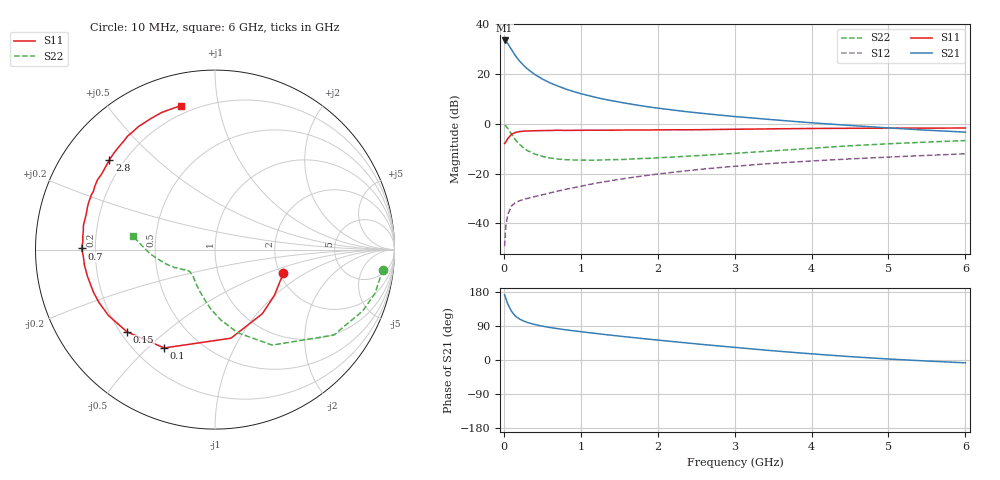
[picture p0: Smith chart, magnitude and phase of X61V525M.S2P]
! SIEMENS Small Signal Semiconductors
! BFP193W
! Si NPN RF Bipolar Junction Transistor in SOT343
! VCE = 1.5 V  IC = 25 mA
! Common Emitter S-Parameters:  April 1994
# GHz  S  MA  R  50
!  f  S11  S21  S12  S22
! GHz  MAG  ANG  MAG  ANG  MAG  ANG  MAG  ANG
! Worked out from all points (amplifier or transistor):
!   40 points, 10 MHz to 6 GHz, reference 50 ohm
!   highest |S21| = 33.5 dB at 10 MHz (marker M1)
!   |S21| within 3 dB of that: start of sweep to 86.36 MHz
!   unconditionally stable (mu >= 1): 783.3 MHz to 4.294 GHz
!   at 200 MHz: K = 0.42, MSG = 28.1 dB, |S12| = -30.9 dB
!   at 1.5 GHz: K = 1.14, MAG = 13.3 dB, |S12| = -22.3 dB
!   at 6 GHz: K = 0.96, MSG = 4.4 dB, |S12| = -12.0 dB
!   S11 on the Smith chart (normalised r, x): 10 MHz: 2.09, -0.66; 100 MHz: 0.32, -0.56; 150 MHz: 0.23, -0.38; 700 MHz: 0.15, +0.00; 2.8 GHz: 0.15, +0.36; 6 GHz: 0.16, +0.78
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0.01  0.4028 -19.1  47.2 172.3  0.0035 86.1  0.9415 -6.8
0.02  0.4178 -37.6  46.48 166.3  0.0068 78.4  0.924 -15.4
0.03  0.444 -53.5  45.17 159.9  0.0098 72.4  0.8912 -22.5
0.05  0.5016 -79.8  41.16 148.2  0.015 63.4  0.8154 -35.7
0.1  0.6167 -117.3  30.9 128.2  0.0224 48.8  0.6202 -59.1
0.15  0.6711 -136.9  23.45 116.0  0.0263 42.0  0.4806 -74.7
0.2  0.6976 -148.1  18.54 108.6  0.0284 39.5  0.3929 -85.3
0.25  0.7104 -155.4  15.3 103.4  0.0302 39.0  0.3364 -93.4
0.3  0.7177 -160.7  12.9 99.6  0.0316 39.0  0.2948 -99.9
0.4  0.726 -168.1  9.845 93.7  0.0345 41.3  0.2481 -109.8
0.5  0.7328 -173.2  7.954 89.3  0.0376 44.0  0.2223 -117.3
0.6  0.7347 -177.2  6.651 85.7  0.041 46.4  0.2062 -123.0
0.7  0.7438 179.5  5.758 82.7  0.0446 48.5  0.1964 -127.3
0.9  0.7404 174.0  4.484 77.2  0.052 52.0  0.1886 -133.4
1.1  0.7452 169.6  3.697 72.3  0.0602 54.1  0.1861 -137.8
1.6  0.7513 159.7  2.57 60.9  0.0812 56.1  0.1941 -143.6
2.2  0.7612 149.4  1.892 48.6  0.1066 55.0  0.2154 -149.8
2.8  0.7721 139.6  1.501 37.0  0.1323 52.1  0.2453 -155.7
3.2  0.7838 133.3  1.323 29.7  0.1485 49.7  0.268 -160.5
4.5  0.8126 116.2  0.928 8.9  0.1977 40.7  0.3628 -176.4
5.5  0.8204 107.5  0.745 -2.7  0.2325 34.3  0.4305 174.2
6  0.8245 103.2  0.682 -7.5  0.2502 31.4  0.4615 170.5
